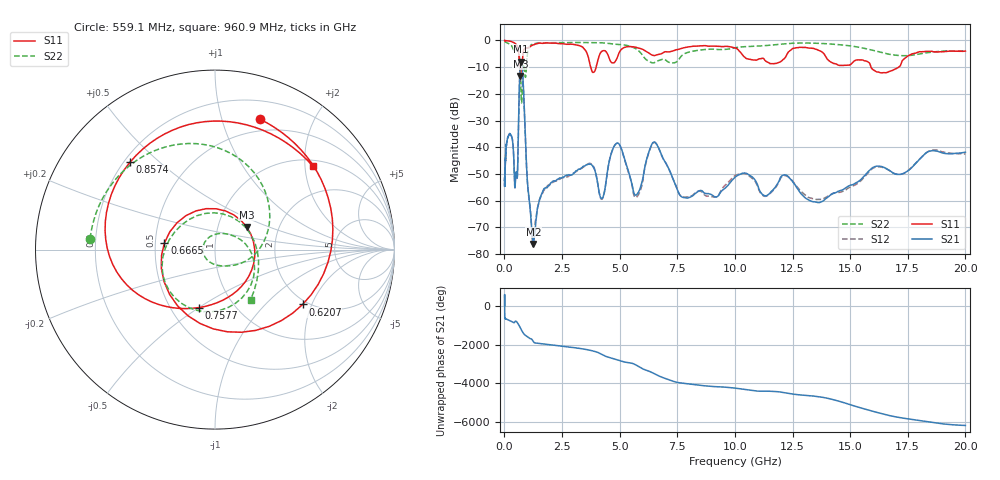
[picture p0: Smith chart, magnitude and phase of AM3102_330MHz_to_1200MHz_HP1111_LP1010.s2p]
! Date/Time: Tue, Sep 11, 2018 5:24 PM
! Network Analyzer: Agilent Technologies E8362B Rev: A.07.50.63
! Sweep from 0.010 to 20.000 GHz, 1601 Points, Sweep Type: LOG
! Power Supply: 4.949 V, 0.001 A
# Hz S DB R 50
!freq MagS11 AngS11 MagS21 AngS21 MagS12 AngS12 MagS22 AngS22
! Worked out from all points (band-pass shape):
!   1601 points, 10 MHz to 20 GHz, reference 50 ohm
!   highest |S21| = -7.89 dB at 729.5 MHz (marker M1); lowest = -76.1 dB at 1.26 GHz (marker M2)
!   |S21| within 3 dB of the highest: 679.8 MHz to 781.5 MHz (101.7 MHz wide, 13.9 % of centre)
!   lowest |S11| = -13.3 dB at 699 MHz (marker M3), VSWR 1.55, Z = 68.6 + j18.2 ohm
!   |S11| at or under -10 dB: 660.3 MHz to 752.8 MHz (92.49 MHz wide, 13.1 % of centre); 3.744 GHz to 3.98 GHz (235.9 MHz wide, 6.11 % of centre); 15.91 GHz to 17.1 GHz (1.196 GHz wide, 7.25 % of centre)
!   |S22| runs from -23.4 to -0.2 dB; largest |S21 - S12| = 0.0047
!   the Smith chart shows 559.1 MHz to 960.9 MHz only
!   S11 on the Smith chart (normalised r, x): 559.1 MHz: 0.38, +1.34; 620.7 MHz: 1.88, -1.72; 666.5 MHz: 0.56, +0.04; 757.7 MHz: 0.69, -0.50; 857.4 MHz: 0.22, +0.41; 960.9 MHz: 1.15, +2.20
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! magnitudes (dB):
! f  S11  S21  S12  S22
! 10 MHz  0.0  -52.5  -53.6  -0.2
! 35.55 MHz  -0.1  -46.5  -46.8  -0.5
! 126.4 MHz  -0.2  -37.0  -37.0  -0.9
! 334.7 MHz  -0.6  -36.5  -36.4  -2.3
! 447.2 MHz  -1.0  -54.3  -54.4  -3.9
! 559.1 MHz  -2.3  -51.2  -51.3  -3.1
! 620.7 MHz  -4.8  -27.9  -28.0  -4.2
! 666.5 MHz  -10.9  -13.2  -13.2  -7.8
! 699 MHz  -13.3  -8.9  -8.9  -13.2
! 729.5 MHz  -12.0  -7.9  -7.9  -21.9
! 757.7 MHz  -9.5  -8.8  -8.9  -22.7
! 857.4 MHz  -3.4  -23.9  -24.0  -9.3
! 960.9 MHz  -2.9  -47.0  -47.2  -9.3
! 1.26 GHz  -1.7  -76.1  -76.0  -1.3
! 1.59 GHz  -1.0  -58.0  -58.1  -0.9
! 4.23 GHz  -4.1  -59.1  -59.4  -0.9
! 4.878 GHz  -6.8  -38.4  -38.5  -1.5
! 5.652 GHz  -2.5  -57.7  -58.5  -2.9
! 6.487 GHz  -5.6  -38.0  -38.2  -8.4
! 7.808 GHz  -2.7  -58.8  -58.7  -5.0
! 13.48 GHz  -3.2  -60.4  -59.4  -1.0
! 20 GHz  -4.0  -41.8  -42.5  -3.9
